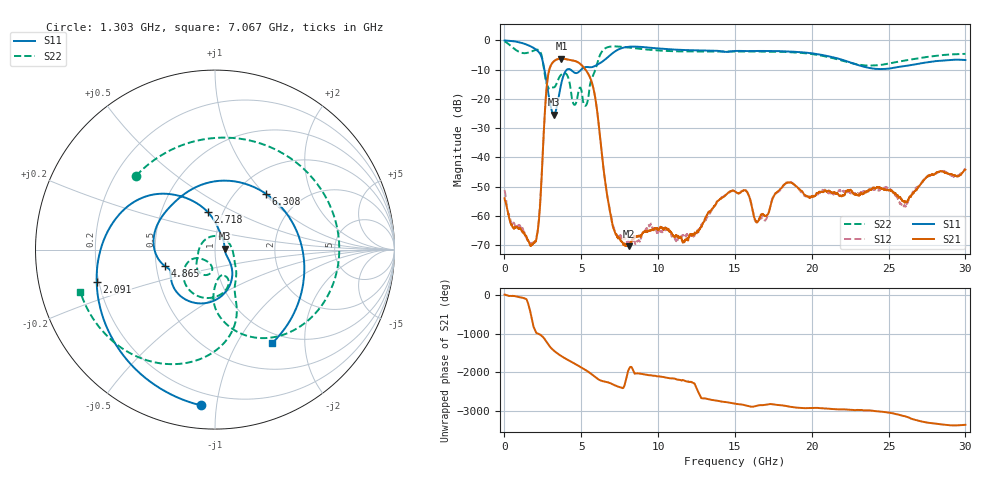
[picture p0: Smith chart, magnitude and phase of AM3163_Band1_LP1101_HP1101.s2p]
!Agilent Technologies,E8364B,MY43040894,A.07.50.67
!Agilent E8364B: A.07.50.67
!Date: Thursday, August 20, 2020 11:20:31
!Correction: S11(Full 2 Port(1,2))
!S21(Full 2 Port(1,2))
!S12(Full 2 Port(1,2))
!S22(Full 2 Port(1,2))
!S2P File: Measurements: S11, S21, S12, S22:
# Hz S  dB  R 50
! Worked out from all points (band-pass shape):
!   3201 points, 10 MHz to 30 GHz, reference 50 ohm
!   highest |S21| = -6.24 dB at 3.712 GHz (marker M1); lowest = -70.4 dB at 8.089 GHz (marker M2)
!   |S21| within 3 dB of the highest: 2.966 GHz to 5.151 GHz (2.185 GHz wide, 53.8 % of centre)
!   lowest |S11| = -25.4 dB at 3.215 GHz (marker M3), VSWR 1.11, Z = 55.7 + j0.556 ohm
!   |S11| at or under -10 dB: 2.602 GHz to 4.072 GHz (1.47 GHz wide, 44 % of centre); 4.292 GHz to 5 GHz (708.1 MHz wide, 15.2 % of centre)
!   |S22| runs from -22.4 to -0.4 dB; largest |S21 - S12| = 0.0042
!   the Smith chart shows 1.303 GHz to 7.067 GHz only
!   S11 on the Smith chart (normalised r, x): 1.303 GHz: 0.13, -0.90; 2.091 GHz: 0.19, -0.13; 2.718 GHz: 0.85, +0.37; 4.865 GHz: 0.56, -0.11; 6.308 GHz: 1.35, +1.02; 7.067 GHz: 0.85, -1.42
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1e7  -0.05 -5.0  -53.99 13.5  -51.14 137.7  -0.40 -14.4
5.067094e8  -0.26 -36.4  -63.67 -18.9  -63.03 -41.0  -2.35 -96.1
1.303319e9  -1.20 -95.3  -65.96 -84.3  -65.73 -83.9  -4.41 136.9
2.090556e9  -3.31 -164.7  -67.53 98.6  -66.94 73.7  -3.20 7.4
2.718472e9  -13.50 100.6  -17.79 -119.3  -17.82 -119.4  -14.25 -89.1
3.215181e9  -25.38 5.3  -7.17 0.2  -7.19 0.2  -16.10 -70.0
3.711891e9  -14.50 -60.2  -6.24 -144.1  -6.27 -144.0  -11.66 -88.0
4.255459e9  -9.90 -131.0  -6.73 90.8  -6.72 90.9  -14.95 -152.9
4.864631e9  -10.69 -161.4  -7.79 -44.7  -7.78 -44.7  -16.49 -108.8
5.014581e9  -9.93 -170.1  -8.47 -79.7  -8.45 -79.7  -17.26 -138.6
5.773703e9  -9.05 120.0  -16.09 77.7  -16.11 77.2  -11.98 -64.2
6.3079e9  -7.51 47.8  -37.34 -61.9  -37.38 -62.0  -4.13 -98.8
7.067022e9  -4.28 -58.5  -63.85 -157.5  -63.19 -156.1  -2.08 -162.5
8.088556e9  -2.20 -153.6  -70.39 -136.2  -68.63 17.5  -2.48 142.6
1.000979e10  -2.80 100.4  -64.72 52.8  -65.67 55.8  -3.47 64.0
1.225904e10  -3.41 10.5  -66.43 -113.6  -66.88 -4.4  -3.85 -14.4
1.5005e10  -3.65 -70.9  -51.69 60.8  -51.72 61.1  -3.82 -92.1
1.64389e10  -3.65 -106.1  -62.22 13.0  -62.02 9.6  -3.83 -127.3
2.000958e10  -4.45 163.3  -53.42 -49.1  -53.44 -53.2  -4.69 136.5
2.274617e10  -8.01 60.8  -52.45 -102.1  -52.43 -102.7  -7.99 21.4
2.500479e10  -9.66 -62.5  -51.22 -168.6  -50.47 -166.2  -7.99 -92.5
3e10  -6.74 104.6  -44.21 -125.6  -43.87 -131.7  -4.63 102.4
